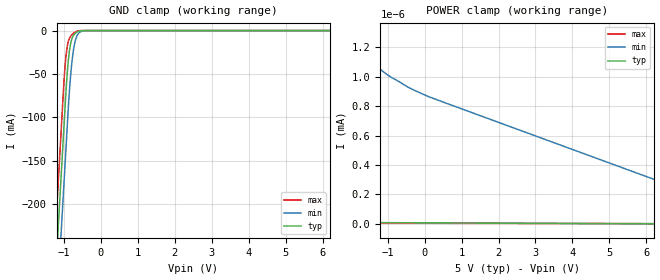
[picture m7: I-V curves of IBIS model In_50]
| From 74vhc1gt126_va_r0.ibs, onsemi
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|//////////////////////////////////////////////////////////////////////////////
|//////////////////////////////////////////////////////////////////////////////
[Model]  In_50
Model_type Input
Vinh = 2.00
Vinl = 0.80
|  variable   typ   min   max
C_comp   2.6pF   2.6pF   2.6pF
|//////////////////////////////////////////////////////////////////////////////
[Temperature Range]   25   125   -55
|//////////////////////////////////////////////////////////////////////////////
[Voltage Range]   5.00V   4.50V   5.50V
|//////////////////////////////////////////////////////////////////////////////
[POWER Clamp Reference] 5.00V   4.50V   5.50V
|//////////////////////////////////////////////////////////////////////////////
[GND Clamp Reference]   0V   0V   0V
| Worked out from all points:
|   GND clamp passes 1 mA (typ) near -0.61 V on its own axis
|   POWER clamp passes 1 mA (typ) near -4.99 V on its own axis
|//////////////////////////////////////////////////////////////////////////////
[GND Clamp]
|   Voltage   I(typ)   I(min)   I(max)
-5V       -3.103A    -3.148A    -3.072A
-1.225V   -279.9mA   -344.5mA   -228.9mA
-1.15V    -223.8mA   -288.8mA   -172.5mA
-1.1V     -186.4mA   -251.6mA   -134.8mA
-1.05V    -149mA     -214.5mA   -97.17mA
-975mV    -92.94mA   -158.8mA   -43.83mA
-925mV    -57.83mA   -121.7mA   -23.05mA
-875mV    -32.25mA   -84.54mA   -11.67mA
-775mV    -8.275mA   -33.13mA   -4.462mA
-650mV    -1.776mA   -6.297mA   -739.6uA
-375mV    -833.1nA   -27.74uA   -20.7nA
10V       11.32pA    1.35nA     5.363pA
|//////////////////////////////////////////////////////////////////////////////
[POWER Clamp]
|   Voltage   I(typ)   I(min)   I(max)
-5V       1.241mA    4.576nA    28.23mA
-4.9V     1.959nA    4.23nA     26.18mA
-4.85V    630.1pA    4.074nA    25.11mA
-4.75V    403.6pA    3.792nA    22.85mA
-4.45V    214.7pA    3.128nA    14.73mA
-4V       95.99pA    2.464nA    78.35uA
-3.95V    88.55pA    2.406nA    138.1pA
-3.65V    54.47pA    2.107nA    19.71pA
-2.25V    10.36pA    1.328nA    4.355pA
-1.1V     7.216pA    1.032nA    3.84pA
100mV     5.954pA    865.9pA    3.302pA
10V       -4.46pA    -47.74pA   -1.133pA
